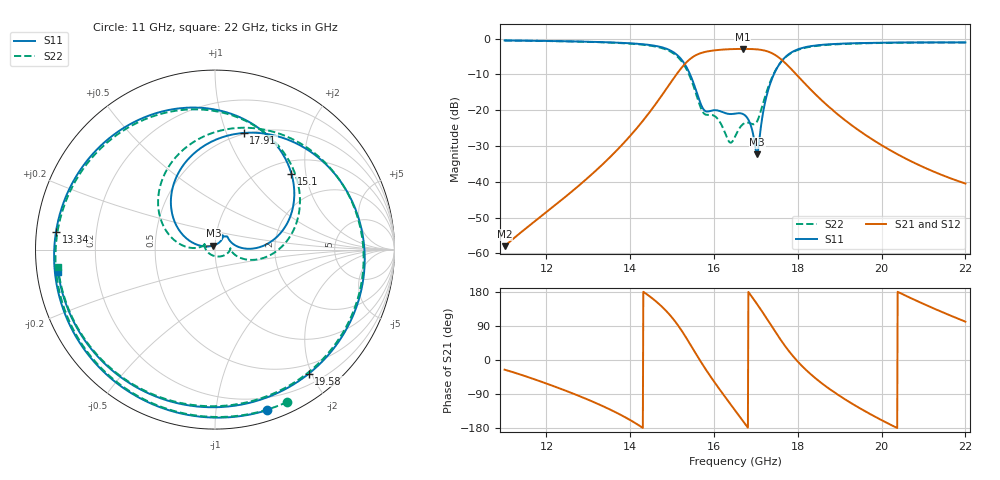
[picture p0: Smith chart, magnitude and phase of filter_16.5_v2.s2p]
! TOUCHSTONE file generated by CST MICROWAVE STUDIO
! Date and time: Fri Apr 08 20:02:04 2016
! Project name: filter_16.5_v2.cst
! Header version: 2015
! Port assignment regex: !\s*Touchstone port\s*([0-9]+)\s*=\s*CST MWS port\s*([0-9]+)\s*\(\"(.*)\"\)(\s*mode\s*([0-9]+))?.*
! Touchstone port assignment:
! Touchstone port 1 = CST MWS port 1 ("")
! Touchstone port 2 = CST MWS port 2 ("")
# GHZ S MA R 50
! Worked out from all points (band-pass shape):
!   1001 points, 11 GHz to 22 GHz, reference 50 ohm
!   highest |S21| = -2.90 dB at 16.69 GHz (marker M1); lowest = -58.0 dB at 11 GHz (marker M2)
!   |S21| within 3 dB of the highest: 15.41 GHz to 17.61 GHz (2.201 GHz wide, 13.3 % of centre)
!   lowest |S11| = -32.3 dB at 17.03 GHz (marker M3), VSWR 1.05, Z = 49.1 + j2.23 ohm
!   |S11| at or under -10 dB: 15.43 GHz to 17.43 GHz (2 GHz wide, 12.2 % of centre)
!   |S22| runs from -29.1 to -0.5 dB; largest |S21 - S12| = 9.4e-05
!   S11 on the Smith chart (normalised r, x): 11 GHz: 0.09, -1.37; 13.34 GHz: 0.06, +0.06; 15.1 GHz: 1.26, +1.66; 17.91 GHz: 0.49, +1.15; 19.58 GHz: 0.35, -1.96; 22 GHz: 0.06, -0.07
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11  0.9406 -72.2  0.001262 -25.5  0.001262 -25.5  0.9394 -64.5
11.891  0.9283 -114.2  0.003369 -57.8  0.003369 -57.8  0.9264 -107.5
12.837  0.9076 -160.3  0.009525 -97.5  0.009525 -97.5  0.9038 -155.4
13.343  0.8915 173.6  0.0176 -121.6  0.0176 -121.6  0.8857 177.0
13.992  0.8592 136.7  0.04338 -158.1  0.04338 -158.1  0.8492 137.4
14.674  0.7753 88.0  0.1383 149.0  0.1383 149.0  0.7569 83.8
15.103  0.6001 44.8  0.3157 97.0  0.3157 97.0  0.5747 35.3
15.411  0.332 9.6  0.5083 45.0  0.5083 45.0  0.3071 -6.0
15.752  0.1021 20.4  0.6434 -16.4  0.6434 -16.4  0.09076 -3.9
16.137  0.0972 48.9  0.6961 -78.2  0.6961 -78.2  0.06873 -21.1
16.5  0.08949 62.1  0.7144 -132.7  0.7144 -132.7  0.04254 -159.6
16.687  0.08853 60.7  0.7165 -160.5  0.7165 -160.5  0.06356 156.5
17.028  0.02421 110.6  0.7059 147.3  0.7059 147.3  0.06992 162.0
17.38  0.2716 145.6  0.6254 88.6  0.6254 88.6  0.2828 160.2
17.633  0.5001 111.0  0.494 46.5  0.494 46.5  0.4968 125.4
17.908  0.6694 76.1  0.342 7.1  0.342 7.1  0.6588 88.8
18.337  0.7877 33.2  0.1861 -40.3  0.1861 -40.3  0.7744 42.9
18.898  0.8413 -9.9  0.09282 -87.2  0.09282 -87.2  0.8297 -3.6
19.58  0.8666 -52.9  0.0465 -133.6  0.0465 -133.6  0.858 -49.7
20.174  0.8773 -85.8  0.02825 -168.6  0.02825 -168.6  0.871 -84.5
21.153  0.884 -134.0  0.0146 140.5  0.0146 140.5  0.88 -134.8
22  0.883 -171.8  0.009453 101.2  0.009453 101.2  0.8801 -173.6
